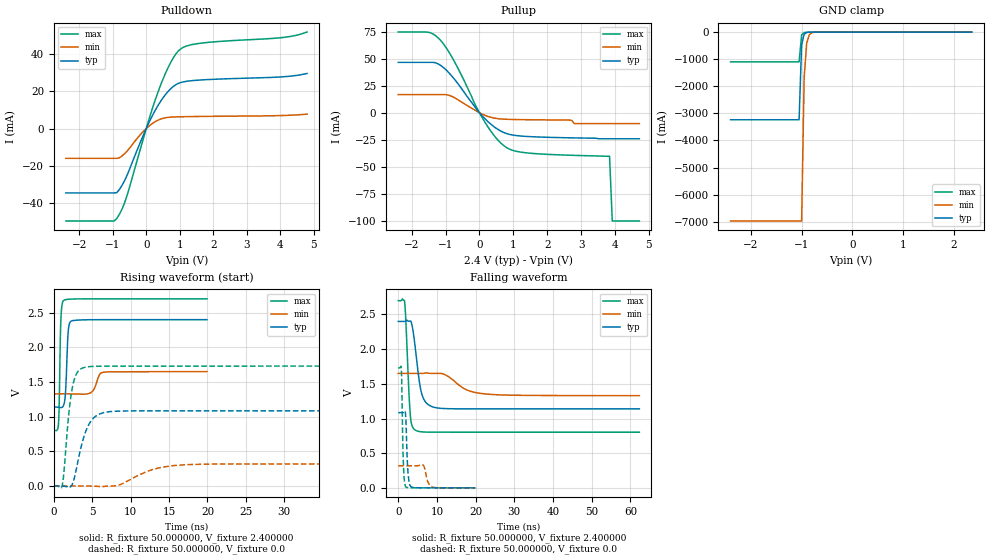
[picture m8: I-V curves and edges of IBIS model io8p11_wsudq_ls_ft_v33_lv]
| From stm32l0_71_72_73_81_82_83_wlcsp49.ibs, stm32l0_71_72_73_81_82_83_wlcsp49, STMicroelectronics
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|   Model io8p11_wsudq_ls_ft_v33_lv
[Model]  io8p11_wsudq_ls_ft_v33_lv
Model_type I/O
Polarity   Non-Inverting
Enable   Active-Low
Vinl =   0.720000V
Vinh =   1.680000V
Vmeas =  1.200000V
Cref =   50.000000pF
Rref =   100.000000M
Vref =   0.0V
C_comp   2.600600pF   2.574200pF   2.601000pF
[Temperature Range]   25.000000   0.125000k   -40.000000
[Pullup Reference]   2.400000V   1.650000V   2.700000V
[Pulldown Reference]   0.0V   0.0V   0.0V
[POWER Clamp Reference]   2.400000V   1.650000V   2.700000V
[GND Clamp Reference]   0.0V   0.0V   0.0V
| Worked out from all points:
|   slope of the pulldown table from 0 to 0.36 V, typ, clamps not added: 28.5 ohm
|   slope of the pullup table from 0 to 0.36 V, typ, clamps not added: 32.2 ohm
|   GND clamp passes 1 mA (typ) near -0.65 V on its own axis
|   rising waveform, R_fixture 50.000000, V_fixture 2.400000: 20-80 % time 279ps typ, 650ps min, 195ps max; typ from 1.14 V to 2.4 V
|   rising waveform, R_fixture 50.000000, V_fixture 0.0: 20-80 % time 1.59ns typ, 4.01ns min, 928ps max; typ from 0 V to 1.08 V
|   falling waveform, R_fixture 50.000000, V_fixture 2.400000: 20-80 % time 1.8ns typ, 5.23ns min, 920ps max; typ from 2.4 V to 1.14 V
|   falling waveform, R_fixture 50.000000, V_fixture 0.0: 20-80 % time 481ps typ, 906ps min, 380ps max; typ from 1.08 V to 0 V
[Pulldown]
|Voltage   I(typ)   I(min)   I(max)
-2.4V     -34.7mA    -16.06mA   -49.82mA
-960mV    -34.7mA    -16.06mA   -49.82mA
-880mV    -34.55mA   -16.06mA   -48.46mA
-720mV    -30.52mA   -14.74mA   -43.28mA
-560mV    -24.65mA   -11.94mA   -35.33mA
0V        0A         0A         142fA
400mV     13.84mA    4.882mA    22.03mA
720mV     21.25mA    6.107mA    35.26mA
1.04V     24.82mA    6.324mA    43.03mA
1.6V      26.11mA    6.486mA    45.88mA
4V        27.76mA    6.965mA    48.87mA
4.8V      29.63mA    7.736mA    51.96mA
[Pullup]
|Voltage   I(typ)   I(min)   I(max)
-2.4V     46.57mA    16.84mA    74.62mA
-1.52V    46.57mA    16.84mA    74.5mA
-1.2V     44.83mA    16.84mA    68.61mA
-720mV    30.24mA    13.64mA    46.11mA
-160mV    6.586mA    2.887mA    9.467mA
160mV     -5.477mA   -2.317mA   -8.695mA
480mV     -14.04mA   -5.139mA   -22.91mA
800mV     -19.2mA    -6.004mA   -32.18mA
1.52V     -22.07mA   -6.444mA   -37.42mA
3.84V     -24mA      -10mA      -40.2mA
3.92V     -24mA      -10mA      -100mA
4.72V     -24mA      -10mA      -100mA
[GND_clamp]
|Voltage   I(typ)   I(min)   I(max)
-2.4V     -3.237A    -6.974A    -1.1A
-1.05V    -3.237A    -6.974A    -1.1A
-1V       -475.9mA   -6.974A    -104.3mA
-950mV    -76.36mA   -1.682A    -18.56mA
-900mV    -16.77mA   -411.9mA   -9.293mA
-850mV    -6.713mA   -104mA     -6.724mA
-800mV    -4.108mA   -28.09mA   -4.924mA
-600mV    -516uA     -827.9uA   -497.3uA
2.35V     0A         0A         0A
[POWER_clamp]
|Voltage   I(typ)   I(min)   I(max)
-2.4V     0A         0A         0A
0V        0A         0A         0A
[Ramp]
| variable   typ   min   max
dV/dt_r  0.65070/1.58340n   0.19118/4.00354n   1.03800/0.92504n
dV/dt_f  0.75690/1.79320n   0.18906/5.22444n   1.13815/0.91691n
R_load = 50.000000
[Rising Waveform]
R_fixture= 50.000000
V_fixture= 2.400000
V_fixture_min= 1.650000
V_fixture_max= 2.700000
|time   V(typ)   V(min)   V(max)
0s        1.139V     1.329V     802.5mV
600.6ps   1.136V     1.329V     888.9mV
680.7ps   1.135V     1.329V     1.093V
920.9ps   1.132V     1.329V     2.405V
1.281ns   1.166V     1.329V     2.678V
1.522ns   1.347V     1.329V     2.689V
1.882ns   2.241V     1.329V     2.694V
2.242ns   2.379V     1.329V     2.697V
6.486ns   2.4V       1.641V     2.7V
19.94ns   2.4V       1.65V      2.7V
[Rising Waveform]
R_fixture= 50.000000
V_fixture= 0.0
V_fixture_min= 0.0
V_fixture_max= 0.0
|time   V(typ)   V(min)   V(max)
0s        -26.59uV   1.012uV    234.2uV
1.126ns   -1.191mV   -12.95uV   25.04mV
2.002ns   -25.53mV   76.42uV    1.096V
2.377ns   16.95mV    80.86uV    1.399V
3.003ns   284.6mV    84.44uV    1.63V
4.004ns   739.8mV    -190.9uV   1.712V
5.38ns    1.001V     -3.421mV   1.727V
8.008ns   1.079V     2.665mV    1.73V
17.39ns   1.085V     308.4mV    1.73V
62.31ns   1.085V     318.6mV    1.73V
[Falling Waveform]
R_fixture= 50.000000
V_fixture= 2.400000
V_fixture_min= 1.650000
V_fixture_max= 2.700000
|time   V(typ)   V(min)   V(max)
0s        2.4V       1.65V      2.7V
1.627ns   2.399V     1.65V      2.698V
1.877ns   2.403V     1.65V      2.512V
2.753ns   2.404V     1.65V      1.392V
3.128ns   2.404V     1.65V      1.047V
4.505ns   1.974V     1.65V      829.6mV
6.131ns   1.345V     1.65V      807.6mV
9.384ns   1.16V      1.651V     802.8mV
22.9ns    1.139V     1.352V     802.5mV
62.31ns   1.139V     1.329V     802.5mV
[Falling Waveform]
R_fixture= 50.000000
V_fixture= 0.0
V_fixture_min= 0.0
V_fixture_max= 0.0
|time   V(typ)   V(min)   V(max)
0s        1.085V     318.6mV    1.73V
800.8ps   1.085V     318.6mV    1.72V
1.161ns   1.084V     318.6mV    709.4mV
1.361ns   1.089V     318.6mV    318.1mV
1.962ns   1V         318.6mV    14.49mV
2.482ns   258.8mV    318.6mV    4.056mV
3.203ns   22.26mV    318.6mV    2.27mV
6.486ns   788.2uV    326.2mV    336.4uV
8.969ns   149.1uV    7.634mV    245.2uV
19.94ns   -26.59uV   1.012uV    234.2uV
